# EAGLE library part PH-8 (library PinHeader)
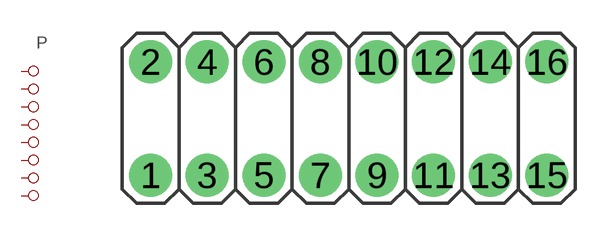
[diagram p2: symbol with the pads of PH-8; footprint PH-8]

Designator prefix P

## PH-8  [PH-8]
1  1  pas
2  1  pas
3  2  pas
4  2  pas
5  3  pas
6  3  pas
7  4  pas
8  4  pas
9  5  pas
10  5  pas
11  6  pas
12  6  pas
13  7  pas
14  7  pas
15  8  pas
16  8  pas

## Footprint PH-8 (pad centres in mm)
drill 1 pad 1.93: 1 -8.89,-2.54; 2 -8.89,2.54; 3 -6.35,-2.54; 4 -6.35,2.54; 5 -3.81,-2.54; 6 -3.81,2.54; 7 -1.27,-2.54; 8 -1.27,2.54; 9 1.27,-2.54; 10 1.27,2.54; 11 3.81,-2.54; 12 3.81,2.54; 13 6.35,-2.54; 14 6.35,2.54; 15 8.89,-2.54; 16 8.89,2.54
